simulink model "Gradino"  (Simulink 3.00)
settings: Solver=ode45  StartTime=0.00  StopTime=1  RelTol=1e-3

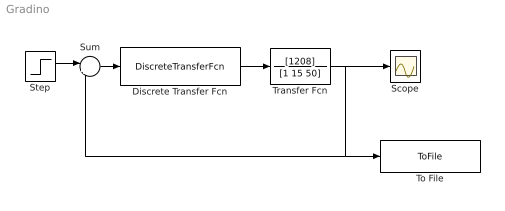
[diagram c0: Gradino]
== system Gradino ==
  Discrete Transfer Fcn : DiscreteTransferFcn  Numerator=[6.335 -12.37 6.046]  Denominator=[1 -1.36 0.36]  SampleTime=0.004
  Scope : Scope
  Step : Step  Time=0.001  Before=0  After=1  SampleTime=0.004
  Sum : Sum  Inputs=|+-  SaturateOnIntegerOverflow=on
  To File : ToFile  Filename=Gradino.mat  MatrixName=Gra  SampleTime=-1
  Transfer Fcn : TransferFcn  Numerator=[1208]  Denominator=[1 15 50]
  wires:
  Sum/1 -> Discrete Transfer Fcn/1
  Discrete Transfer Fcn/1 -> Transfer Fcn/1
  Step/1 -> Sum/1
  Transfer Fcn/1 -> Scope/1, Sum/2, To File/1
